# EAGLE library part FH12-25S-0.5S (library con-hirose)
0.5mm Pitch Connectors For FPC/FFC Source: Data sheet
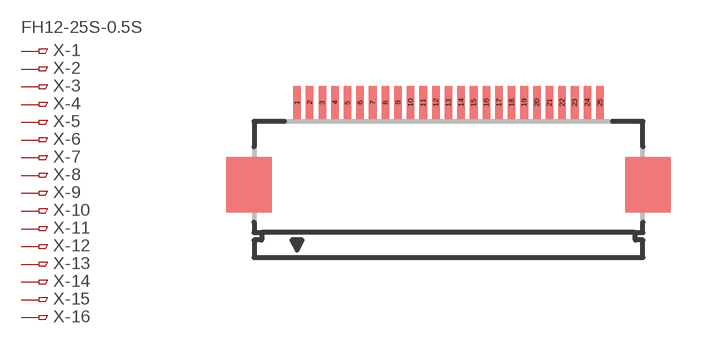
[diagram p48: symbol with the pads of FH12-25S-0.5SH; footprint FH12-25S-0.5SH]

Designator prefix X; gates -1=PINV -2=PIN -3=PIN -4=PIN -5=PIN -6=PIN -7=PIN -8=PIN -9=PIN -10=PIN -11=PIN -12=PIN -13=PIN -14=PIN -15=PIN -16=PIN -17=PIN -18=PIN -19=PIN -20=PIN -21=PIN -22=PIN -23=PIN -24=PIN -25=PIN

## FH12-25S-0.5SH (OC_FARNELL: unknown; OC_NEWARK: unknown)  [FH12-25S-0.5SH]
1  -1:1  pas
2  -2:1  pas
3  -3:1  pas
4  -4:1  pas
5  -5:1  pas
6  -6:1  pas
7  -7:1  pas
8  -8:1  pas
9  -9:1  pas
10  -10:1  pas
11  -11:1  pas
12  -12:1  pas
13  -13:1  pas
14  -14:1  pas
15  -15:1  pas
16  -16:1  pas
17  -17:1  pas
18  -18:1  pas
19  -19:1  pas
20  -20:1  pas
21  -21:1  pas
22  -22:1  pas
23  -23:1  pas
24  -24:1  pas
25  -25:1  pas

## Footprint FH12-25S-0.5SH (pad centres in mm)
0.5mm Pitch Connectors For FPC/FFC Source: Data sheet
smd 0.3 x 1.3: 1 -6,3.25; 2 -5.5,3.25; 3 -5,3.25; 4 -4.5,3.25; 5 -4,3.25; 6 -3.5,3.25; 7 -3,3.25; 8 -2.5,3.25; 9 -2,3.25; 10 -1.5,3.25; 11 -1,3.25; 12 -0.5,3.25; 13 0,3.25; 14 0.5,3.25; 15 1,3.25; 16 1.5,3.25; 17 2,3.25; 18 2.5,3.25; 19 3,3.25; 20 3.5,3.25; 21 4,3.25; 22 4.5,3.25; 23 5,3.25; 24 5.5,3.25; 25 6,3.25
